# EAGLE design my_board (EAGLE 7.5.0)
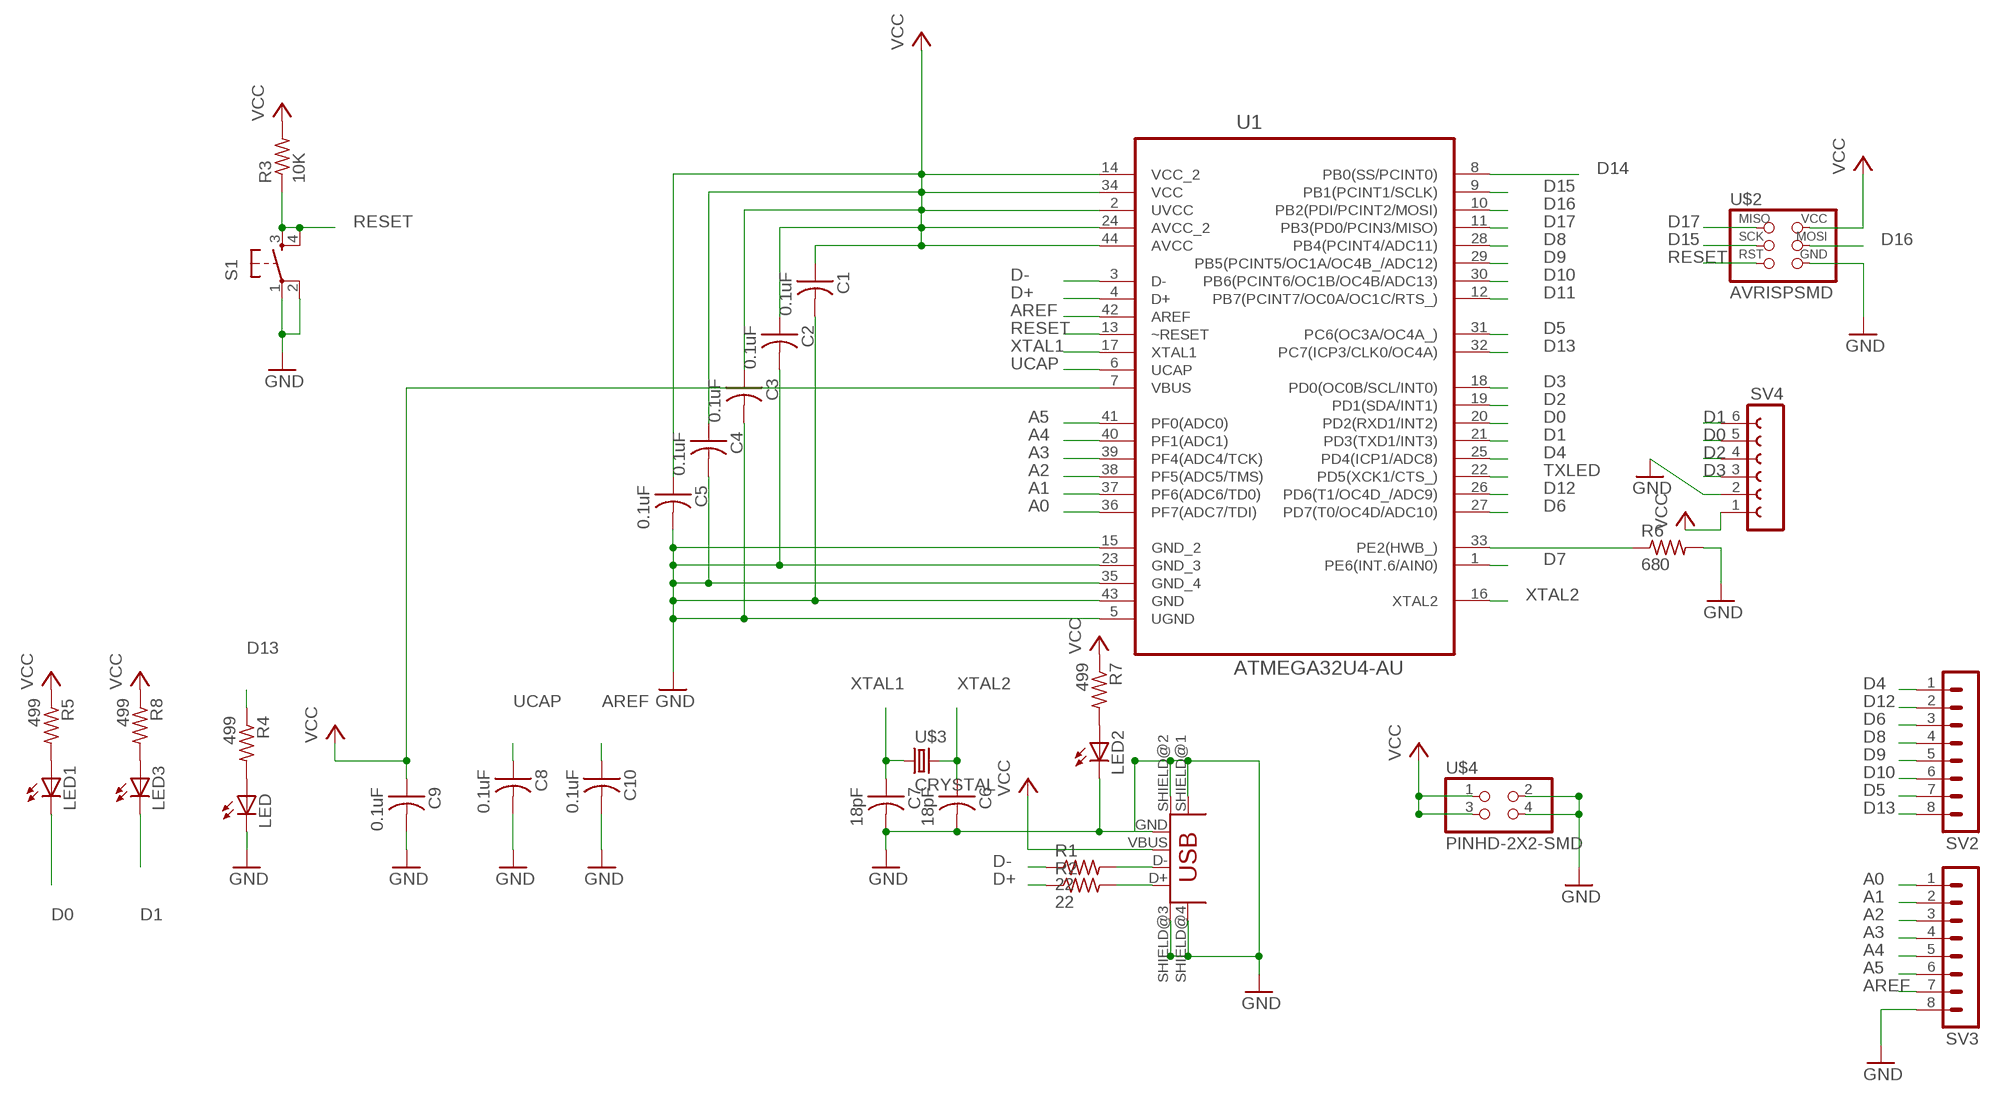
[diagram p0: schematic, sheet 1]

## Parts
C1  0.1uF  CAP-US1206FAB  [C1206FAB]
C2  0.1uF  CAP-US1206FAB  [C1206FAB]
C3  0.1uF  CAP-US1206FAB  [C1206FAB]
C4  0.1uF  CAP-US1206FAB  [C1206FAB]
C5  0.1uF  CAP-US1206FAB  [C1206FAB]
C6  18pF  CAP-US1206FAB  [C1206FAB]
C7  18pF  CAP-US1206FAB  [C1206FAB]
C8  0.1uF  CAP-US1206FAB  [C1206FAB]
C9  0.1uF  CAP-US1206FAB  [C1206FAB]
C10  0.1uF  CAP-US1206FAB  [C1206FAB]
LED  LED1206  [1206]
LED1  LED1206  [1206]
LED2  LED1206  [1206]
LED3  LED1206  [1206]
R1  22  RES-US1206FAB  [R1206FAB]
R2  22  RES-US1206FAB  [R1206FAB]
R3  10K  RES-US1206FAB  [R1206FAB]
R4  499  RESISTOR1206  [1206]
R5  499  RESISTOR1206  [1206]
R6  680  RES-US1206FAB  [R1206FAB]
R7  499  RESISTOR1206  [1206]
R8  499  RESISTOR1206  [1206]
S1  6MM_SWITCH6MM_SWITCH  [6MM_SWITCH]
SV2  MA08-1  [MA08-1]
SV3  MA08-1  [MA08-1]
SV4  FE06-1  [FE06]
U1  ATMEGA32U4-AU  [QFP80P1200X1200X120-44N]
U$1  USB_MINIB  [USB_MINIB]
U$2  AVRISPSMD  [2X03SMD]
U$3  CRYSTAL  [2-SMD-5X3MM]
U$4  PINHD-2X2-SMD  [2X02SMD]

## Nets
A0: SV3.1 U1.36(PF7(ADC7/TDI))
A1: SV3.2 U1.37(PF6(ADC6/TD0))
A2: SV3.3 U1.38(PF5(ADC5/TMS))
A3: SV3.4 U1.39(PF4(ADC4/TCK))
A4: SV3.5 U1.40(PF1(ADC1))
A5: SV3.6 U1.41(PF0(ADC0))
AREF: C10.1 SV3.7 U1.42(AREF)
D0: LED1.2(C) SV4.5 U1.20(PD2(RXD1/INT2))
D1: LED3.2(C) SV4.6 U1.21(PD3(TXD1/INT3))
D2: SV4.4 U1.19(PD1(SDA/INT1))
D3: SV4.3 U1.18(PD0(OC0B/SCL/INT0))
D4: SV2.1 U1.25(PD4(ICP1/ADC8))
D5: SV2.7 U1.31(PC6(OC3A/OC4A_))
D6: SV2.3 U1.27(PD7(T0/OC4D/ADC10))
D7: U1.1(PE6(INT.6/AIN0))
D8: SV2.4 U1.28(PB4(PCINT4/ADC11))
D9: SV2.5 U1.29(PB5(PCINT5/OC1A/OC4B_/ADC12))
D10: SV2.6 U1.30(PB6(PCINT6/OC1B/OC4B/ADC13))
D11: U1.12(PB7(PCINT7/OC0A/OC1C/RTS_))
D12: SV2.2 U1.26(PD6(T1/OC4D_/ADC9))
D13: R4.1 SV2.8 U1.32(PC7(ICP3/CLK0/OC4A))
D14: U1.8(PB0(SS/PCINT0))
D15: U1.9(PB1(PCINT1/SCLK)) U$2.3(SCK)
D16: U1.10(PB2(PDI/PCINT2/MOSI)) U$2.4(MOSI)
D17: U1.11(PB3(PD0/PCIN3/MISO)) U$2.1(MISO)
D+: R2.1 U1.4(D+)
D-: R1.1 U1.3(D-)
GND: C1.2 C2.2 C3.2 C4.2 C5.2 C6.2 C7.2 C8.2 C9.2 C10.2 LED2.2(C) LED.2(C) R6.2 S1.1(P) S1.2(P1) SV3.8 SV4.2 U1.5(UGND) U1.15(GND_2) U1.23(GND_3) U1.35(GND_4) U1.43(GND) U$1.GND U$1.SHIELD@1(SHIELD) U$1.SHIELD@2(SHIELD1) U$1.SHIELD@3(SHIELD2) U$1.SHIELD@4(SHIELD3) U$2.6(GND) U$4.2 U$4.4
N$1: R1.2 U$1.D-
N$2: R2.2 U$1.D+
N$3: LED.1(A) R4.2
N$4: LED1.1(A) R5.2
N$5: LED2.1(A) R7.2
N$6: LED3.1(A) R8.2
N$35: R6.1 U1.33(PE2(HWB_))
RESET: R3.1 S1.3(S) S1.4(S1) U1.13(~RESET) U$2.5(RST)
TXLED: U1.22(PD5(XCK1/CTS_))
UCAP: C8.1 U1.6(UCAP)
VCC: C1.1 C2.1 C3.1 C4.1 C5.1 C9.1 R3.2 R5.1 R7.1 R8.1 SV4.1 U1.2(UVCC) U1.7(VBUS) U1.14(VCC_2) U1.24(AVCC_2) U1.34(VCC) U1.44(AVCC) U$1.VBUS U$2.2(VCC) U$4.1 U$4.3
XTAL1: C7.1 U1.17(XTAL1) U$3.P$1
XTAL2: C6.1 U1.16(XTAL2) U$3.P$2

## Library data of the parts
C1-C10 = fab:CAP-US
LED LED1-LED3 = ng:LED
R1-R3 R6 = fab:RES-US: Resistor (US Symbol)
R4 R5 R7 R8 = ng:RESISTOR
S1 = ng:6MM_SWITCH: OMRON SWITCH
SV2 SV3 = con-lstb:MA08-1: PIN HEADER; OC_FARNELL: unknown; OC_NEWARK: unknown
SV4 = con-lsta:FE06-1: FEMALE HEADER; OC_FARNELL: unknown; OC_NEWARK: unknown
U1 = Atmel_By_element14_Batch_1:ATMEGA32U4-AU: 8-bit Microcontroller with ISP Flash and USB Controller; MPN: ATMEGA32U4-AU; OC_FARNELL: 1748525; OC_NEWARK: 26R5633; PACKAGE: TQFP-44; SUPPLIER: Atmel
U$1 = fab:USB_MINIB
U$2 = fab:AVRISP
U$3 = fab:CRYSTAL
U$4 = fab:PINHD-2X2-SMD

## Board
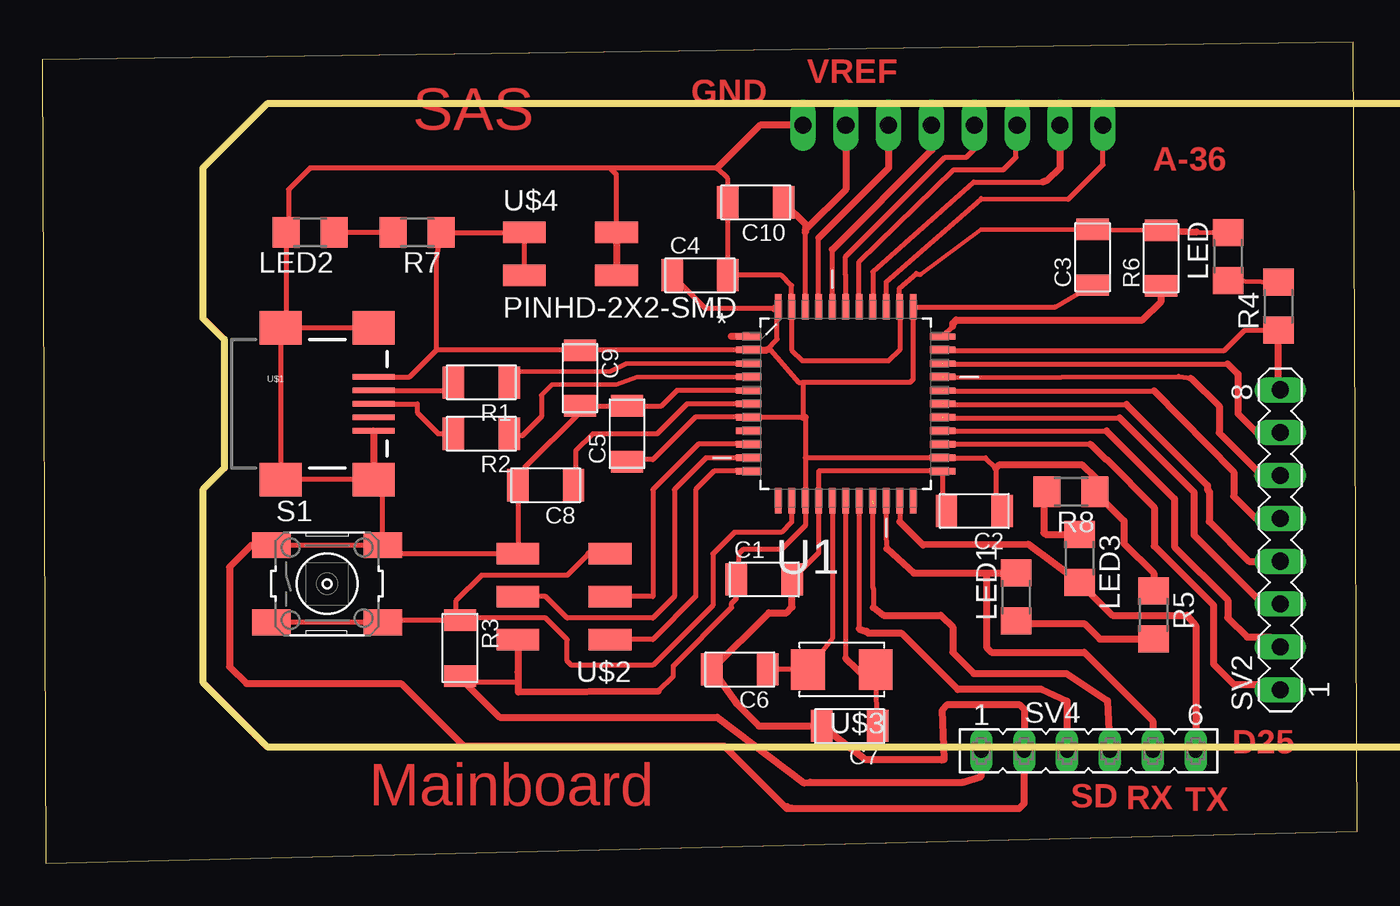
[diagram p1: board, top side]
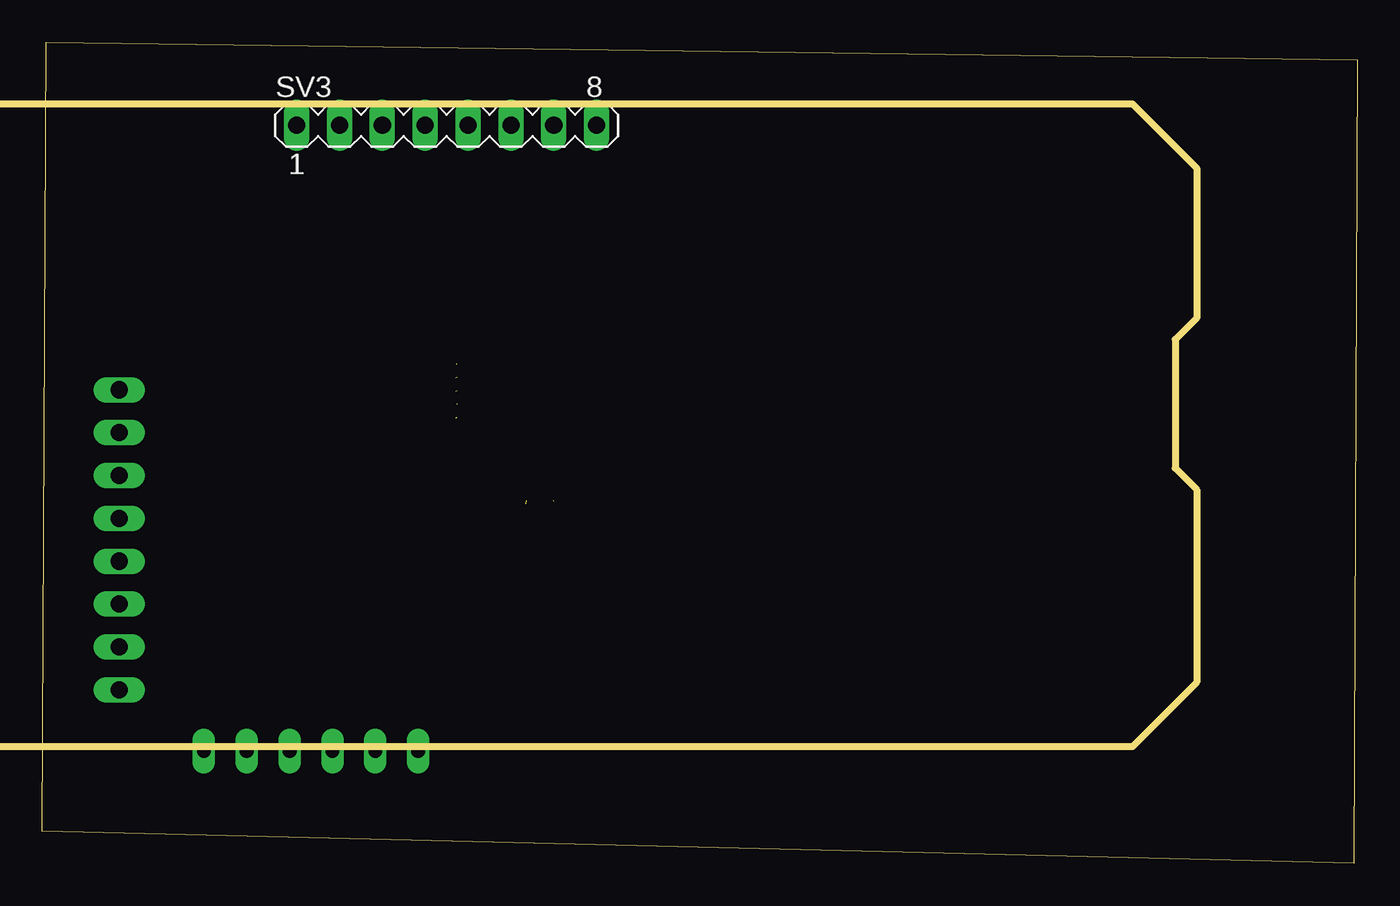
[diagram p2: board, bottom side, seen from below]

Size 77.94 x 48.68 mm. Coordinates in mm from the lower left corner, seen from the top.
Outline: 0.2,0 77.94,1.9 77.69,48.68 0,47.63 0.2,0
Copper layers (1*16): Top 0.035mm / dielectric 1.5mm / Bottom 0.035mm
Design rules "default *": minimum track width 10mil, minimum drill 24mil, track to track 0.4mm, track to pad 0.4mm, pad to pad 0.4mm, via to via 0.4mm, smd to smd 0.4mm, copper to edge 40mil, drill to drill 0.4mm, minimum pad ring 10mil, minimum via ring 8mil, stop-mask expansion 4mil, vias tented up to drill 0mil, thermal gap 10mil
Milling: area 9.5,6.9 to 109.8,45

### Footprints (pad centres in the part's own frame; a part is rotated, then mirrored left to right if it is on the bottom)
C1206FAB = smd 1.27 x 1.905: 1 -1.651,0; 2 1.651,0
1206 = smd 1.6 x 1.803: 1 -1.422,0; 2 1.422,0
R1206FAB = smd 1.27 x 1.905: 1 -1.651,0; 2 1.651,0
6MM_SWITCH = smd 2.286 x 1.524: 1 -3.302,2.286; 2 3.302,2.286; 3 -3.302,-2.286; 4 3.302,-2.286
MA08-1 = drill 1.016 long: 1 -8.89,0; 2 -6.35,0; 3 -3.81,0; 4 -1.27,0; 5 1.27,0; 6 3.81,0; 7 6.35,0; 8 8.89,0
FE06 = drill 0.813 long: 1 -6.35,0; 2 -3.81,0; 3 -1.27,0; 4 1.27,0; 5 3.81,0; 6 6.35,0
QFP80P1200X1200X120-44N = smd 1.5 x 0.38: 1 -5.74,3.988; 2 -5.74,3.2; 3 -5.74,2.388; 4 -5.74,1.6; 5 -5.74,0.787; 6 -5.74,0; 7 -5.74,-0.787; 8 -5.74,-1.6; 9 -5.74,-2.388; 10 -5.74,-3.2; 11 -5.74,-3.988; 23 5.74,-3.988; 24 5.74,-3.2; 25 5.74,-2.388; 26 5.74,-1.6; 27 5.74,-0.787; 28 5.74,0; 29 5.74,0.787; 30 5.74,1.6; 31 5.74,2.388; 32 5.74,3.2; 33 5.74,3.988 | smd 0.38 x 1.5: 12 -3.988,-5.74; 13 -3.2,-5.74; 14 -2.388,-5.74; 15 -1.6,-5.74; 16 -0.787,-5.74; 17 0,-5.74; 18 0.787,-5.74; 19 1.6,-5.74; 20 2.388,-5.74; 21 3.2,-5.74; 22 3.988,-5.74; 34 3.988,5.74; 35 3.2,5.74; 36 2.388,5.74; 37 1.6,5.74; 38 0.787,5.74; 39 0,5.74; 40 -0.787,5.74; 41 -1.6,5.74; 42 -2.388,5.74; 43 -3.2,5.74; 44 -3.988,5.74
USB_MINIB = smd 2.5 x 0.35: D+ 3.77,0; D- 3.77,0.8; GND 3.77,-1.6; ID 3.77,-0.8; VBUS 3.77,1.6 | smd 2.5 x 2: SHIELD@1 -1.73,-4.5; SHIELD@2 -1.73,4.5; SHIELD@3 3.77,4.5; SHIELD@4 3.77,-4.5
2X03SMD = smd 2.54 x 1.27: 1 -2.54,2.54; 2 2.92,2.54; 3 -2.54,0; 4 2.92,0; 5 -2.54,-2.54; 6 2.92,-2.54
2-SMD-5X3MM = smd 2 x 2.4: P$1 -2,0; P$2 2,0
2X02SMD = smd 2.54 x 1.27: 1 -2.54,1.27; 2 2.92,1.27; 3 -2.54,-1.27; 4 2.92,-1.27

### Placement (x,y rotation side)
C1  42.79,16.83 0 top
C2  55.24,20.89 180 top
C3  62.26,35.93 90 top
C4  38.98,34.86 0 top
C5  34.67,25.46 90 top
C6  41.34,11.49 180 top
C7  47.85,8.14 180 top
C8  29.84,22.41 180 top
C9  31.87,28.76 270 top
C10  42.29,39.18 180 top
LED  70.27,35.98 90 top
LED1  57.73,15.79 90 top
LED2  15.87,37.4 180 top
LED3  61.48,18.08 270 top
R1  26.03,28.51 180 top
R2  26.03,25.46 180 top
R3  24.76,12.76 270 top
R4  73.27,33.03 90 top
R5  65.87,14.72 270 top
R6  66.31,35.88 90 top
R7  22.22,37.4 180 top
R8  60.97,22.02 180 top
S1  16.89,16.57 0 top
SV2  73.38,19.18 90 top
SV3  53.97,43.75 0 bottom
SV4  62.01,6.66 0 top
U1  47.62,27.24 0 top
U$1  15.87,27.24 0 top
U$2  31.11,15.81 180 top
U$3  47.39,11.49 180 top
U$4  31.11,36.13 0 top

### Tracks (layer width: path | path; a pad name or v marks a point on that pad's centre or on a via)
A0
  Top 0.305: SV3.1 62.86,41.41 60.81,39.36 55.66,39.41 50.01,34.46 U1.36
A1
  Top 0.305: 59.3,40.39 55.19,40.39 49.22,35.07 U1.37
  Top 0.406: SV3.2 60.32,41.21 59.55,40.48 59.3,40.39
A2
  Top 0.305: U1.38 48.41,35.66 54.01,41.11 56.96,41.11 57.71,41.86 57.71,42.96 57.76,43.01 57.76,42.91 57.78,42.93 SV3.3
A3
  Top 0.305: U1.39 47.62,33.6 47.61,33.61 47.61,34.85 47.62,34.86 47.61,34.87 47.61,35.96 53.51,41.86 54.76,41.86 55.24,42.34 55.24,43.01
  Top 0.406: 55.24,42.48 55.24,43.01 SV3.4 | 55.29,43.31 55.29,44.05
A4
  Top 0.305: U1.40 46.83,36.39
  Top 0.406: SV3.5 52.7,42.26 46.83,36.39
A5
  Top 0.305: U1.41 46.02,37.07
  Top 0.406: SV3.6 50.16,41.21 46.02,37.07
AREF
  Top 0.305: U1.42 45.23,37.4
  Top 0.406: C10.1 45.23,37.88 45.23,37.55 | SV3.7 47.62,39.94 45.23,37.55 | 45.23,37.55 45.23,37.4
D0
  Top 0.305: U1.20 50.01,19.31 50.06,18.66
  Top 0.406: 50.06,18.66 51.66,17.21 55.96,17.21 | 55.96,17.21 LED1.2 | 55.96,17.21 55.96,12.81 56.26,12.51 61.76,12.51 65.82,8.45 SV4.5
D1
  Top 0.305: U1.21 50.82,20.25
  Top 0.406: SV4.6 68.36,14.11 67.86,14.71 63.43,14.71 LED3.2 58.43,18.91 52.21,18.86 50.82,20.25
D2  (1 unrouted)
  Top 0.305: 49.26,21.31 49.21,21.26 49.21,16.36 49.26,16.31 49.26,15.16
  Top 0.406: 49.26,15.16 49.86,14.71 53.26,14.71 53.96,14.01 53.96,12.51 55.21,11.26 60.71,11.26 63.13,9.64 SV4.4
D3
  Top 0.305: U1.18 48.41,13.91
  Top 0.406: 48.41,13.91 48.86,13.76 48.96,13.66 50.91,13.66 54.26,10.31 59.26,10.31 60.74,9.63 SV4.3
D4
  Top 0.305: U1.25 62.12,24.85
  Top 0.406: 62.12,24.85 63.01,23.96 63.06,23.96 65.91,21.11 65.91,18.81 69.41,15.31 69.41,11.81 70.61,10.61 73.06,10.61 SV2.1
D5  (1 unrouted)
  Top 0.305: 53.38,29.61 70.26,29.61
  Top 0.406: 70.26,29.61 70.86,29.01 70.86,26.66 71.99,25.53 SV2.7
D6  (1 unrouted)
  Top 0.305: 53.4,26.41 63.86,26.41
  Top 0.406: 63.86,26.41 68.26,22.01 68.26,19.46 72.35,15.37 SV2.3
D7
  Top 0.406: U1.1 40.84,31.23
D8  (1 unrouted)
  Top 0.305: 53.39,27.26 53.44,27.21 64.26,27.21
  Top 0.406: 64.26,27.21 69.06,22.41 69.06,22.16 69.16,22.06 69.16,20.26 71.51,17.91 SV2.4
D9  (1 unrouted)
  Top 0.305: 53.43,28.01 65.91,28.01
  Top 0.406: 65.91,28.01 70.61,23.21 70.61,21.76 71.92,20.45 SV2.5
D10  (1 unrouted)
  Top 0.305: 53.44,28.81 67.36,28.86 68.06,28.76
  Top 0.406: 72.03,22.99 SV2.6 72.28,22.99 69.76,25.51 69.76,27.11 68.06,28.76
D12
  Top 0.305: U1.26 63.08,25.64
  Top 0.406: 63.08,25.64 67.11,21.61 67.11,18.76 70.26,15.61 70.26,14.56 71.41,13.41 72.8,13.41 SV2.2
D13
  Top 0.305: U1.32 53.39,30.41 70.06,30.41 71.26,31.61 R4.1
  Top 0.406: SV2.8 73.27,28.18 R4.1
D15
  Top 0.305: U1.9 38.88,24.85 36.19,22.16 36.19,15.81 U$2.3
D16
  Top 0.305: U1.10 39.34,24.04 37.46,22.16 37.46,15.81 36.19,14.54 31.11,14.54 29.84,15.81 U$2.4
D17
  Top 0.305: U1.11 39.82,23.25 38.73,22.16 38.73,15.81 36.19,13.27 U$2.1
D+
  Top 0.254: U1.4 35.25,28.84 34.03,28.38 30.22,28.38 29.59,27.75
  Top 0.305: 29.59,27.75 29.59,26.48 28.44,25.34 27.81,25.34 R2.1
D-
  Top 0.254: U1.3 34.64,29.63 33.65,29.14 27.81,29.14
  Top 0.305: 27.81,29.14 27.55,28.64 R1.1
GND
  Top 0.254: 52.06,34.91 55.63,37.58 C3.2
  Top 0.305: S1.1 S1.2 20.19,22.19 | U$1.SHIELD@4 U$1.SHIELD@1 U$1.SHIELD@2 U$1.SHIELD@3 | U1.5 37.61,28.03 36.7,27.11 C5.2 C9.2 | LED2.2 14.45,32.05 | C3.2 R6.2 | 68.4,37.42 LED.2 | 53.36,21.12 U1.23 46.02,23.25 U1.15 46.02,18.4 C1.2 | U$2.6 20.19,18.35 | C8.2 U$2.6 | 33.65,41.21 40,41.21 40.63,40.58 C10.2 C4.2 43.81,34.86 44.42,34.25 U1.43 44.42,30.44 45.08,29.78 50.16,29.78 50.82,30.44 U1.35 50.81,32.99 50.81,34.11 51.81,34.96 52.06,34.91 | 33.65,41.21 15.87,41.21 14.6,39.94 14.6,37.55 | U$4.4 34.03,40.83 33.65,41.21 | 31.87,26.73 28.57,23.43 28.57,22.79
  Top 0.406: U$1.GND U$1.SHIELD@4 20.19,22.19 | U$1.SHIELD@3 19.68,31.74 | 14.45,32.05 U$1.SHIELD@2 | R6.2 68.4,37.42 | 53.36,21.12 C2.2 | 20.19,18.35 S1.2 | U$4.2 U$4.4 | C9.2 31.87,26.73 | 28.57,22.79 C8.2 | U$2.6 | 44.45,16.45 C1.2 44.45,15.2 44.11,14.86 43.06,14.86 C6.2 41.14,9.48 42.48,8.14 C7.2 48.78,6.16 53.46,6.16 | 14.6,37.55 LED2.2 | SV3.8 42.54,43.75 40,41.21 | S1.1 12.41,18.86 11.11,17.56 11.11,11.66 12.11,10.66 21.26,10.66 24.96,6.96 40.41,6.96 44.01,3.36 | 53.46,6.16 53.31,6.11 | 53.46,6.16 53.36,9.11 53.66,9.41 57.91,9.41 58.2,9.12 58.2,7.16 | 58.21,7.67 58.2,7.16 | 58.2,7.16 SV4.2 58.2,3.55 57.91,3.26 44.11,3.26 44.01,3.36 | 44.01,3.36 44.16,3.36 44.16,3.26 44.46,3.26
N$1
  Top 0.305: U$1.D- 24.38,28.04
  Top 0.406: 24.38,28.04 R1.2
N$2
  Top 0.305: R2.2 23.49,25.46 22.22,26.73 22.22,27.24 U$1.D+
N$3
  Top 0.305: LED.1 R4.2
N$4
  Top 0.406: LED1.1 57.89,14.21 61.76,14.21 62.67,13.3 R5.2
N$5
  Top 0.305: R7.2 LED2.1
N$6
  Top 0.406: R8.2 59.36,21.83 59.36,19.61 59.46,19.51 LED3.1
N$35
  Top 0.305: 53.96,31.83 U1.33
  Top 0.406: 53.96,31.83 53.96,32.01 54.16,32.21 65.21,32.21 66.31,33.31 R6.1
RESET
  Top 0.305: S1.4 S1.3 | U1.13 44.42,20.23 43.81,19.62 41.02,19.62 39.75,18.35 39.75,15.3 36.19,11.75 31.36,11.75 31.11,12 31.11,13.27 29.84,14.54 24.89,14.54 | 32.38,18.35 31.11,17.08 26.03,17.08 24.51,15.56 24.51,14.67 R3.1 20.19,14.41
  Top 0.406: 24.89,14.54 R3.1 | U$2.5 32.38,18.35 | 20.19,14.41 S1.4
UCAP
  Top 0.305: U1.6 38.22,27.24 36.44,25.46 32.63,25.46 31.62,24.45 31.62,22.54 C8.1
VCC
  Top 0.305: 42.95,30.44 43.56,31.05 43.56,32.9 | 31.9,30.44 U1.2 43.15,30.44 44.83,28.51 45.08,28.51 | C9.1 23.36,30.41 | 23.36,30.41 21.79,28.84 U$1.VBUS | 23.36,30.41 23.36,35.85 R7.1 U$4.1 U$4.3 | C3.1 60.04,32.98 U1.34 51.61,28.69 51.43,28.51 45.08,28.51 | 56.51,21.27 56.51,23.43 55.9,24.04 U1.24 45.23,24.04 | 43.38,32.88 39.31,32.88 C4.1 | 41.27,16.95 41.27,18.35 41.52,18.6 43.81,18.6 45.23,20.03 U1.14 45.23,24.04 | 45.23,26.45 45.23,24.04 | 45.08,28.51 45.08,26.45 U1.7 38.7,26.45 36.19,23.94 34.28,23.94 C5.1 | R3.2 25.1,10.77 28.2,10.77 | 36.51,10.21 37.41,11.11 37.41,11.71 40.86,15.16 40.86,15.41 41.14,15.69 C1.1
  Top 0.406: U1.2 42.95,30.44 | 43.56,32.9 U1.44 43.38,32.88 | 51.68,32.9 U1.34 | 31.9,30.44 C9.1 | 37.46,34.73 C4.1 | 56.51,21.27 C2.1 | 41.27,16.95 C1.1 41.21,16.76 | 45.08,26.45 45.23,26.45 | 56.51,23.43 56.69,23.61 61.66,23.61 62.44,22.83 R8.1 64.11,20.3 64.11,18.96 65.87,17.2 R5.1 | 55.71,7.61 SV4.1 55.66,5.16 54.56,4.81 45.51,4.81 45.16,4.76 40.01,8.66 27.11,8.66 24.71,11.06 R3.2 | 36.51,10.21 28.21,10.16 28.2,10.77 28.19,11.33 U$2.2
XTAL1  (1 unrouted)
  Top 0.305: C7.1 49.41,10.98 U$3.P$1 | 47.61,21.46 47.61,12.16
  Top 0.406: 47.61,12.16 48.84,10.98 49.41,10.98
XTAL2
  Top 0.305: C6.1 U$3.P$2 46.83,13.33 U1.16

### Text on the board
Top: VREF | GND | SAS | A-36 | D25 | Mainboard | SD | RX | TX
